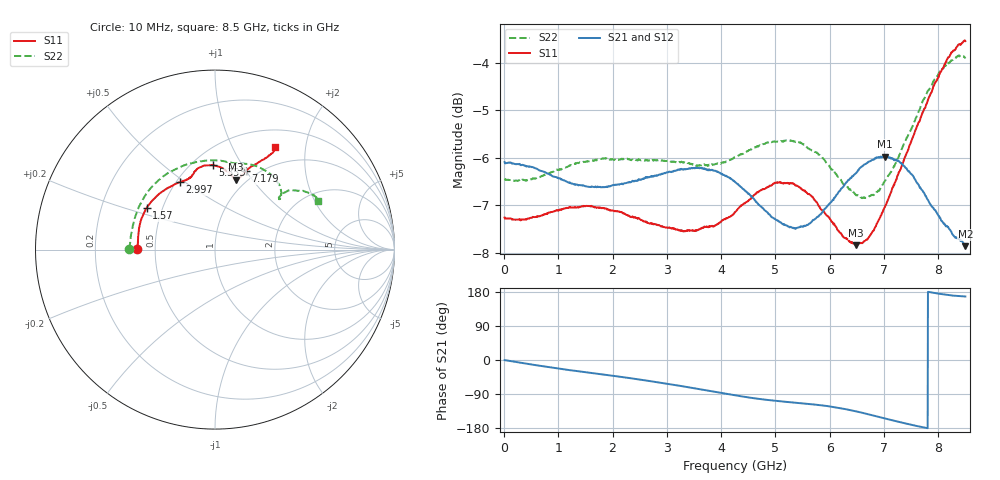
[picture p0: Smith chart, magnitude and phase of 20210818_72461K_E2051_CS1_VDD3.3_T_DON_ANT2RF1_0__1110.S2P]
!Agilent Technologies,E5071C,MY46417908,A.11.23
!Date: Wed Aug 18 14:23:45 2021
!Data & Calibration Information:
!Freq	S11:SOLT2(ON)	S21:SOLT2(ON)	S12:SOLT2(ON)	S22:SOLT2(ON)
!PortZ  Port1:50+j0  Port2:50+j0
!Above PortZ is port z conversion or system Z0 setting when saving the data.
!When reading, reference impedance value at option line is always used.
# Hz S dB R 50
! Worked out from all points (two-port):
!   1601 points, 10 MHz to 8.5 GHz, reference 50 ohm
!   highest |S21| = -5.97 dB at 7.014 GHz (marker M1); lowest = -7.9 dB at 8.5 GHz (marker M2)
!   |S21| within 3 dB of the highest: start of sweep to end of sweep
!   lowest |S11| = -7.8 dB at 6.489 GHz (marker M3), VSWR 2.36, Z = 44.7 + j41.6 ohm
!   |S11| at or under -10 dB: nowhere
!   |S22| runs from -6.8 to -3.9 dB; largest |S21 - S12| = 0.0026
!   S11 on the Smith chart (normalised r, x): 10 MHz: 0.39, +0.00; 1.57 GHz: 0.41, +0.24; 2.997 GHz: 0.52, +0.48; 5.353 GHz: 0.63, +0.76; 7.179 GHz: 0.89, +0.99; 8.5 GHz: 0.73, +1.49
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1e7  -7.26 179.7  -6.09 -0.4  -6.09 -0.4  -6.44 179.6
7.847125e8  -7.17 165.7  -6.32 -18.2  -6.32 -18.2  -6.35 156.1
1.426769e9  -7.02 151.9  -6.58 -30.8  -6.58 -30.8  -6.09 135.5
1.570038e9  -7.01 148.6  -6.61 -33.5  -6.62 -33.5  -6.07 130.7
2.190869e9  -7.17 133.8  -6.56 -45.3  -6.56 -45.3  -6.03 110.9
2.843538e9  -7.42 120.2  -6.36 -59.1  -6.36 -59.1  -6.05 93.9
2.997419e9  -7.47 117.4  -6.31 -62.6  -6.30 -62.6  -6.07 90.6
3.655394e9  -7.47 109.7  -6.22 -78.4  -6.22 -78.4  -6.16 79.9
4.255e9  -7.15 105.8  -6.51 -93.1  -6.50 -93.2  -5.99 72.7
4.759094e9  -6.66 101.3  -7.05 -103.7  -7.05 -103.7  -5.72 65.0
5.353394e9  -6.56 91.3  -7.48 -112.5  -7.49 -112.4  -5.66 52.6
5.671769e9  -6.82 84.9  -7.34 -116.8  -7.36 -116.7  -5.85 46.3
6.170556e9  -7.54 76.7  -6.71 -126.5  -6.73 -126.6  -6.41 39.5
6.488931e9  -7.84 73.5  -6.32 -135.6  -6.33 -135.8  -6.79 38.0
6.722406e9  -7.67 71.8  -6.08 -143.7  -6.08 -143.8  -6.82 38.4
7.01425e9  -7.04 69.9  -5.97 -154.2  -5.98 -154.2  -6.49 39.5
7.088538e9  -6.84 69.5  -5.99 -156.8  -6.00 -156.8  -6.37 39.7
7.178744e9  -6.57 68.7  -6.03 -159.9  -6.03 -159.9  -6.18 39.8
7.502425e9  -5.66 64.9  -6.34 -171.0  -6.34 -171.0  -5.40 38.0
7.842025e9  -4.70 61.1  -6.95 179.1  -6.93 179.0  -4.55 33.3
8.213462e9  -3.86 59.1  -7.51 170.9  -7.48 171.0  -4.00 28.0
8.5e9  -3.55 59.6  -7.86 167.5  -7.81 167.4  -3.92 25.3
